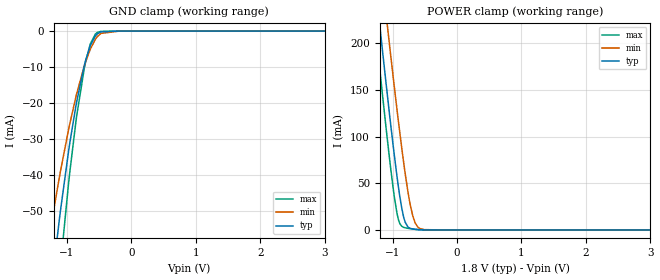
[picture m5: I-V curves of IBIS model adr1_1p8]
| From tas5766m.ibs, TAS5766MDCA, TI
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|   adr1_1p8 Model
[Model]   adr1_1p8
Model_type   Input
Vinl = 0.54
Vinh = 1.26
|   typ   min   max
|   (nom PVT)   (fast PVT)   (slow PVT)
C_comp   6.950e-12   6.878e-12   7.098e-12
[Model spec]
|subparameter
Vinl   0.54   0.486   0.594
Vinh   1.26   1.134   1.386
| Where nom  PVT is Nominal Process, 1.8V, 27C
|   Fast PVT is Strong Process,  1.98V, -40C
|   Slow PVT is Weak Process,   1.62V, 125C
[Voltage Range]   1.8   1.62   1.98
|Junction Temperature
[Temperature Range]   27   125   -40
[Power Clamp Reference]   1.8   1.62   1.98
[GND Clamp Reference]   0   0   0
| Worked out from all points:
|   GND clamp passes 1 mA (typ) near -0.54 V on its own axis
|   POWER clamp passes 1 mA (typ) near -0.68 V on its own axis
[GND Clamp]
|   Voltage   I(typ)   I(min)   I(max)
-1.8V     -258.5mA   -159.1mA   -368.5mA
-1.248V   -72.95mA   -54.75mA   -97.42mA
-1.223V   -69.04mA   -52.09mA   -91.95mA
-1.099V   -50.31mA   -39.24mA   -65.8mA
-972.4mV  -33.61mA   -27.55mA   -42.63mA
-952.2mV  -31.2mA    -25.83mA   -39.31mA
-845.6mV  -19.69mA   -17.47mA   -23.63mA
-726.8mV  -9.566mA   -9.704mA   -10.32mA
-633.8mV  -4.034mA   -5.019mA   -3.573mA
-527.4mV  -781.1uA   -1.581mA   -409.5uA
-180mV    -19.22nA   -796.1nA   0A
3.6V      0A         0A         0A
[POWER Clamp]
|   Voltage   I(typ)   I(min)   I(max)
-1.8V     623.7mA    688.3mA    587.1mA
-1.403V   354.1mA    425.1mA    310.3mA
-1.189V   213.4mA    287.1mA    166.4mA
-1.099V   156mA      230.4mA    108.5mA
-1.051V   126.5mA    200.8mA    79.19mA
-931.7mV  57.79mA    129.3mA    18.15mA
-829.8mV  14.42mA    73.33mA    2.878mA
-761.6mV  3.259mA    41.06mA    1.751mA
-683.3mV  1.014mA    14.39mA    940.4uA
-607.7mV  454.3uA    3.109mA    396.2uA
-508.9mV  103.8uA    361.3uA    59.98uA
3.6V      0A         0A         0A
